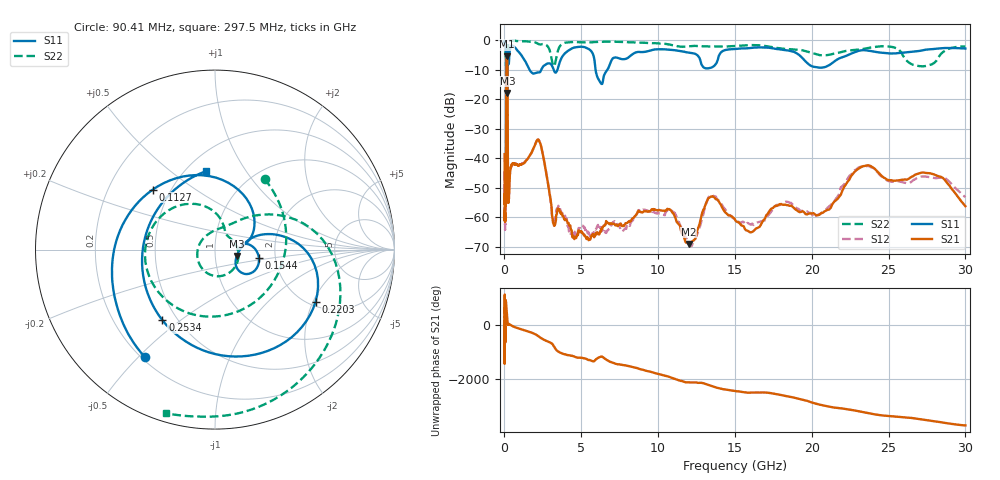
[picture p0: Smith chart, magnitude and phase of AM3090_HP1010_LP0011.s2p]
! Date/Time: Thu, Feb 28, 2019 2:04 PM
! Network Analyzer: Agilent Technologies E8364B Rev: A.07.50.67
! Sweep from 0.010 to 30.000 GHz, 1601 Points, Sweep Type: LOG
! Power Supply: 5.023 V, 0.002 A
# Hz S DB R 50
!freq MagS11 AngS11 MagS21 AngS21 MagS12 AngS12 MagS22 AngS22
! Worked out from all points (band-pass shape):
!   1601 points, 10 MHz to 30 GHz, reference 50 ohm
!   highest |S21| = -5.59 dB at 155.2 MHz (marker M1); lowest = -69.1 dB at 12.01 GHz (marker M2)
!   |S21| within 3 dB of the highest: 126.5 MHz to 191.4 MHz (64.98 MHz wide, 40.9 % of centre)
!   lowest |S11| = -18.0 dB at 186.8 MHz (marker M3), VSWR 1.29, Z = 63.6 - j4.68 ohm
!   |S11| at or under -10 dB: 1.624 GHz to 2.401 GHz (776.4 MHz wide, 38.6 % of centre); 3.201 GHz to 3.454 GHz (253.6 MHz wide, 7.62 % of centre); 5.927 GHz to 6.71 GHz (782.7 MHz wide, 12.4 % of centre)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
!   |S22| runs from -20.9 to -0.2 dB; largest |S21 - S12| = 0.013
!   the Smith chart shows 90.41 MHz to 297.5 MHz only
!   S11 on the Smith chart (normalised r, x): 90.41 MHz: 0.21, -0.52; 112.7 MHz: 0.40, +0.35; 154.4 MHz: 1.64, -0.17; 220.3 MHz: 2.18, -2.09; 253.4 MHz: 0.42, -0.43; 297.5 MHz: 0.62, +0.67
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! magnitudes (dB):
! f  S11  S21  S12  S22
! 10 MHz  -0.3  -38.6  -44.5  -0.5
! 38.04 MHz  -0.5  -58.4  -61.0  -1.4
! 48.61 MHz  -0.7  -50.1  -48.7  -1.5
! 90.41 MHz  -2.9  -53.1  -52.7  -6.4
! 112.7 MHz  -6.3  -21.5  -21.5  -8.1
! 144.7 MHz  -13.9  -5.7  -5.7  -18.7
! 154.4 MHz  -12.1  -5.6  -5.6  -16.7
! 155.2 MHz  -12.0  -5.6  -5.6  -16.6
! 186.8 MHz  -18.0  -7.5  -7.5  -19.7
! 202.3 MHz  -10.8  -15.4  -15.4  -10.8
! 220.3 MHz  -4.0  -44.1  -44.1  -2.7
! 253.4 MHz  -6.2  -54.3  -54.2  -0.8
! 297.5 MHz  -7.1  -52.6  -51.8  -0.4
! 550.5 MHz  -2.1  -41.9  -42.0  -0.2
! 2.084 GHz  -11.1  -34.3  -34.3  -1.0
! 3.22 GHz  -10.3  -62.7  -61.6  -8.9
! 7.926 GHz  -6.3  -62.1  -64.0  -0.7
! 12.01 GHz  -4.3  -69.1  -69.3  -2.1
! 13.54 GHz  -9.2  -52.9  -52.6  -2.2
! 20.41 GHz  -9.3  -59.3  -59.2  -5.0
! 23.48 GHz  -3.5  -42.6  -42.8  -2.9
! 30 GHz  -2.9  -56.3  -53.2  -2.2
